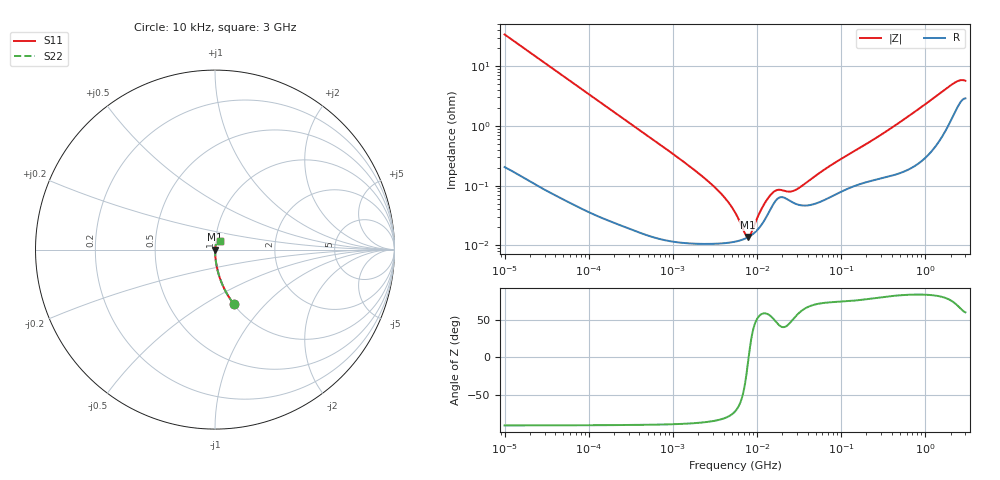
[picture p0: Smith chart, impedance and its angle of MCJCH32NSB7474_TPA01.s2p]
! MCJCH32NSB7474_TPA01  S-PARAMETER MODEL  ( Standard Model )
! Model Generated by TAIYO YUDEN Corporation (http://www.ty-top.com)
! Version 1.0
! TAIYO YUDEN Control No. 220601
! Copyright(c) 2015 TAIYO YUDEN CO.,LTD. All Rights Reserved.
! Product Description (link to TY-COMPAS)
! https://ds.yuden.co.jp/TYCOMPAS/or/detail?pn=MCJCH32NSB7474KTPA01&u=M
! Products Name : Multilayer Ceramic Capacitors
! Characteristics :
!  Capacitance : 0.47 [uF] , Rated Voltage : 100 [V] , TCC : X7R
!  Case Size : 3.2 x 2.5 / 0.126 x 0.098 [mm/inch] , Thickness : 1.9 / 0.075 [mm/inch]
!  (Conditions: Temperature = 25 [degC] , DC Bias Voltage = 0 [V])
! External Node Assignments :
!  1  o---| |---o  2
! GND o---------o GND
! Frequency Range : 10kHz  -  3GHz  [ 401 STEP ]
# MHZ S RI R 50
! Freq[MHz].  S11 Real  S11 Imag  S21 Real  S21 Imag  S12 Real  S12 Imag  S22 Real  S22 Imag
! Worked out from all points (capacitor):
!   401 points, 10 kHz to 3 GHz, reference 50 ohm
!   read as one part in series: C = 471 nF near 10.65 kHz
!   lowest |Z| = 13.8 mohm at 7.748 MHz (marker M1)
!   series resonance near 7.95 MHz, so ESL is about 850 pH
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0.01  0.1037 -0.3018  0.8963 0.3018  0.8963 0.3018  0.1037 -0.3018
0.026575  0.0169 -0.1252  0.9831 0.1252  0.9831 0.1252  0.0169 -0.1252
0.082683  0.0021 -0.0411  0.9979 0.0411  0.9979 0.0411  0.0021 -0.0411
0.683653  0.000154 -0.00501  0.9998 0.00501  0.9998 0.00501  0.000154 -0.00501
2.824956  0.000107 -0.00108  0.9999 0.00108  0.9999 0.00108  0.000107 -0.00108
4.124064  0.00011 -0.000622  0.9999 0.000622  0.9999 0.000622  0.00011 -0.000622
5.477226  0.000116 -0.00034  0.9999 0.00034  0.9999 0.00034  0.000116 -0.00034
7.048603  0.000128 -0.00011  0.9999 0.00011  0.9999 0.00011  0.000128 -0.00011
7.747855  0.000136 -2.35e-05  0.9999 2.35e-05  0.9999 2.35e-05  0.000136 -2.35e-05
8.516475  0.000147 6.38e-05  0.9999 -6.38e-05  0.9999 -6.38e-05  0.000147 6.38e-05
10.29003  0.000187 0.000246  0.9998 -0.000246  0.9998 -0.000246  0.000187 0.000246
12.04705  0.000253 0.000406  0.9997 -0.000406  0.9997 -0.000406  0.000253 0.000406
15.50326  0.00048 0.000603  0.9995 -0.000603  0.9995 -0.000603  0.00048 0.000603
18.15044  0.000625 0.000581  0.9994 -0.000581  0.9994 -0.000581  0.000625 0.000581
23.35767  0.000582 0.000541  0.9994 -0.000541  0.9994 -0.000541  0.000582 0.000541
27.34599  0.000513 0.000641  0.9995 -0.000641  0.9995 -0.000641  0.000513 0.000641
45.28751  0.000484 0.00124  0.9995 -0.00124  0.9995 -0.00124  0.000484 0.00124
79.88199  0.00068 0.0022  0.9993 -0.0022  0.9993 -0.0022  0.00068 0.0022
374.4521  0.0015 0.00861  0.9985 -0.00861  0.9985 -0.00861  0.0015 0.00861
2120.803  0.0162 0.0468  0.9838 -0.0468  0.9838 -0.0468  0.0162 0.0468
2562.461  0.0257 0.0499  0.9743 -0.0499  0.9743 -0.0499  0.0257 0.0499
3000  0.0302 0.0461  0.9698 -0.0461  0.9698 -0.0461  0.0302 0.0461
